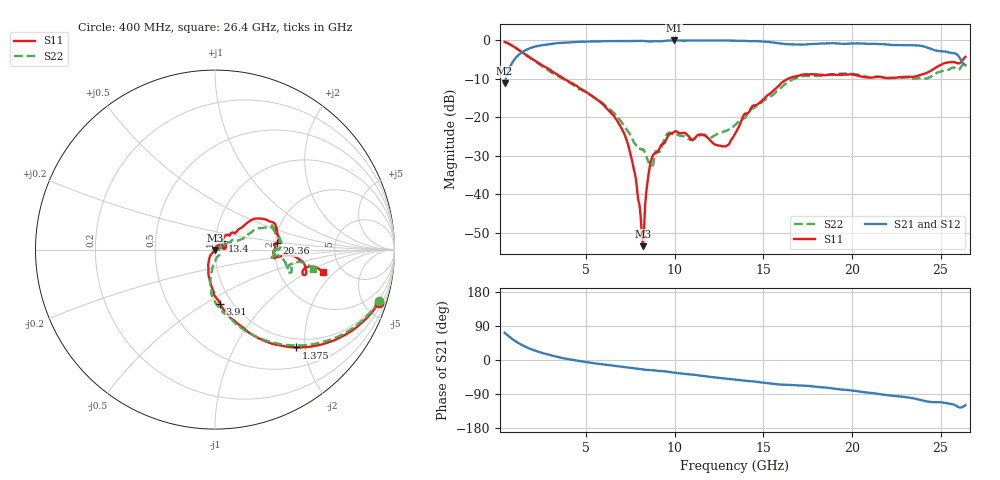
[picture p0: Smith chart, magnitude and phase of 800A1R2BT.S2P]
!  American Technical Ceramics  Date:  12/17/08
!  One Norden Lane
!  Huntington Station,  NY.  11746-2102
!  Tel:  (631) 622-4700  Fax:  (631) 622-4748
!  Part Number  800A1R2BT
!  Description: Broardband capacitor  Mounting Orientation: Vertical
!  Application:
# GHZ S DB R 50
! Freq  |S11|  S11 Ph  |S21|  S21 Ph  |S12|  S12 Ph  |S22|  S22 Ph
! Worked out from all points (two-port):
!   401 points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, 400 MHz to 26.4 GHz, reference 50 ohm
!   highest |S21| = 0.00 dB at 9.955 GHz (marker M1); lowest = -11.2 dB at 400 MHz (marker M2)
!   |S21| within 3 dB of the highest: 1.401 GHz to 25.39 GHz (23.99 GHz wide, 179 % of centre)
!   lowest |S11| = -53.5 dB at 8.2 GHz (marker M3), VSWR 1.00, Z = 49.8 - j0.15 ohm
!   |S11| at or under -10 dB: 3.77 GHz to 16.37 GHz (12.6 GHz wide, 125 % of centre)
!   |S22| runs from -32.8 to -0.4 dB; largest |S21 - S12| = 0.0057
!   S11 on the Smith chart (normalised r, x): 400 MHz: 0.84, -6.22; 1.375 GHz: 0.83, -1.82; 3.91 GHz: 0.88, -0.58; 13.4 GHz: 1.08, +0.10; 20.36 GHz: 2.05, +0.17; 26.4 GHz: 3.55, -1.42
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0.4  -0.36 -18.0  -11.15 72.1  -11.18 72.1  -0.37 -17.3
1.375  -3.00 -50.4  -3.08 39.6  -3.11 39.7  -3.06 -49.5
2.415  -6.17 -68.3  -1.30 20.1  -1.32 20.1  -6.39 -69.8
3.91  -10.39 -84.7  -0.55 3.0  -0.57 3.1  -10.58 -89.4
4.755  -12.70 -92.2  -0.32 -3.7  -0.33 -3.5  -12.87 -94.9
7.095  -23.72 -120.5  -0.15 -18.5  -0.15 -18.3  -21.87 -95.5
7.68  -33.20 -126.6  -0.15 -21.7  -0.14 -21.4  -26.34 -80.1
8.07  -45.32 -103.7  -0.14 -23.7  -0.13 -23.5  -28.16 -55.2
8.2  -53.46 -135.0  -0.11 -24.8  -0.09 -24.6  -28.20 -50.0
8.655  -31.31 57.2  -0.26 -26.8  -0.24 -26.5  -31.97 -18.2
9.11  -28.43 43.7  -0.22 -28.8  -0.21 -28.6  -29.00 18.9
9.955  -23.80 28.9  0.00 -33.3  -0.01 -33.0  -24.36 27.6
12.75  -27.47 22.9  -0.01 -48.3  -0.01 -48.3  -23.67 35.2
13.4  -24.24 49.5  -0.08 -51.6  -0.07 -51.6  -21.97 30.0
13.985  -18.96 44.9  -0.09 -54.7  -0.07 -54.6  -20.13 27.4
16.13  -10.65 36.3  -0.91 -65.2  -0.89 -65.2  -11.72 26.2
17.755  -8.76 19.7  -0.91 -69.6  -0.89 -69.7  -9.22 21.1
20.355  -9.18 6.1  -0.77 -82.8  -0.74 -82.9  -8.89 0.8
22.11  -9.75 -2.7  -1.12 -93.4  -1.10 -93.6  -9.72 -1.6
23.8  -9.06 -6.8  -1.34 -104.7  -1.33 -105.0  -9.78 -8.2
25.945  -5.92 -15.4  -3.70 -122.7  -3.68 -123.0  -7.53 -16.5
26.4  -4.26 -11.8  -6.42 -119.0  -6.41 -119.3  -5.10 -11.1
